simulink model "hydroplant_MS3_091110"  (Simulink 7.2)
settings: Solver=ode23tb  StartTime=0.0  StopTime=1000  MaxStep=0.1  RelTol=1e-4
undefined symbols (not defined in the file or in its folder): Blackbox_Base_sf, sigbuilder_block

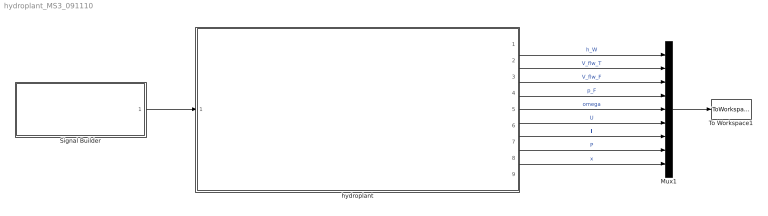
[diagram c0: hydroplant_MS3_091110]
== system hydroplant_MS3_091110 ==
  Mux1 : Mux  Inputs=9
  Signal Builder : Subsystem  Tag=STV Subsys  LoadFcn=sigbuilder_block('load');  StartFcn=sigbuilder_block('start');  StopFcn=sigbuilder_block('stop');  ClipboardFcn=sigbuilder_block('clipboard');
  To Workspace1 : ToWorkspace  VariableName=daten  SampleTime=-1  SaveFormat=Structure With Time
  hydroplant : Subsystem
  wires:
  Signal Builder/1(u) -> hydroplant/1(u)
  Mux1/1 -> To Workspace1/1
  hydroplant/1(h_W) -> Mux1/1  "h_W"
  hydroplant/2(V_flw_T) -> Mux1/2  "V_flw_T"
  hydroplant/3(V_flw_F) -> Mux1/3  "V_flw_F"
  hydroplant/4(p_F) -> Mux1/4  "p_F"
  hydroplant/5(omega) -> Mux1/5  "omega"
  hydroplant/6(U) -> Mux1/6  "U"
  hydroplant/7(I) -> Mux1/7  "I"
  hydroplant/8(P) -> Mux1/8  "P"
  hydroplant/9(x) -> Mux1/9  "x"

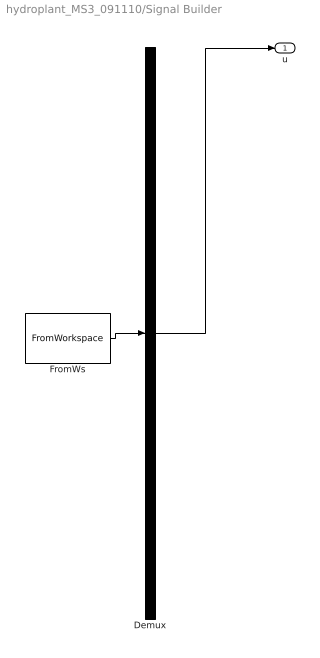
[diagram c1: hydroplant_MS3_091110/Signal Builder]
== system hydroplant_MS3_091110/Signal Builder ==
  Demux : Demux  Tag=STV Demux  Outputs=1
  FromWs : FromWorkspace  Tag=STV FromWs  VariableName=tuvar  SampleTime=0  SigBuilderData=DataTag0  VnvData=DataTag1
  u : Outport  Tag=STV Outport  OutDataType=sfix(16)  OutScaling=2^0
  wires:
  Demux/1 -> u/1
  FromWs/1 -> Demux/1

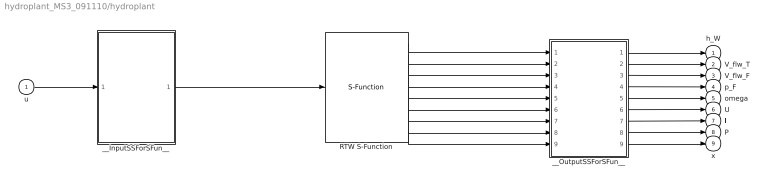
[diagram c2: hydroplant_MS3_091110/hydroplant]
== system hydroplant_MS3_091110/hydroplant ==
  u : Inport  OutDataType=sfix(16)  OutScaling=2^0
  RTW S-Function : S-Function  FunctionName=Blackbox_Base_sf  SFunctionModules=""  EnableBusSupport=off  mask{rtw_sf_name=Blackbox_Base_sf, showVar=off}
      mask prompts: rtw_sf_name "Generated S-function name (model_sf):"; showVar "Show module list"
      mask help: Real-Time Workshop generated S-function.
      mask init:
      | displist = '';
      | if ~strcmp(get_param(gcb, 'FunctionName'), rtw_sf_name);
      |   set_param(gcb, 'FunctionName', rtw_sf_name);
      | end
      | % Check if we are generating RTW code
      | rtw_mode = false;
      | if strcmpi(get_param(bdroot(gcb),'SimulationStatus'),'Initializing')
      | 	rtw_mode = strcmpi(get_param(bdroot(gcb),'BuildingRTWCode'),'on') && ...
      | 		~strcmpi(get_param(bdroot(gcb),'TargetStyle'),'SimulationTarget');
      | end
      | if showVar || rtw_mode
      | 	if exist('rtwsfunc') == 2 | exist('rtwsfunc') == 6
      | 		tmplist = rtwsfunc(rtw_sf_name,gcb);
      | 		tmplist = ['\nList of Modules:\n', tmplist];
      | 	elseif showVar
      | 		tmplist = '\nList of Modules:\nRTW not licensed\n';
      |  	end
      | end
      | if showVar
      |   displist = tmplist;
      | end
  __InputSSForSFun__ : Subsystem
  __OutputSSForSFun__ : Subsystem
  h_W : Outport  PortDimensions=1  SampleTime=[-1 0]  DataType=double  OutDataType=sfix(16)  OutScaling=2^0  OutDataTypeStr=double
  V_flw_T : Outport  Port=2  PortDimensions=1  SampleTime=[-1 0]  DataType=double  OutDataType=sfix(16)  OutScaling=2^0  OutDataTypeStr=double
  V_flw_F : Outport  Port=3  PortDimensions=1  SampleTime=[-1 0]  DataType=double  OutDataType=sfix(16)  OutScaling=2^0  OutDataTypeStr=double
  p_F : Outport  Port=4  PortDimensions=1  SampleTime=[-1 0]  DataType=double  OutDataType=sfix(16)  OutScaling=2^0  OutDataTypeStr=double
  omega : Outport  Port=5  PortDimensions=1  SampleTime=[-1 0]  DataType=double  OutDataType=sfix(16)  OutScaling=2^0  OutDataTypeStr=double
  U : Outport  Port=6  PortDimensions=1  SampleTime=[-1 0]  DataType=double  OutDataType=sfix(16)  OutScaling=2^0  OutDataTypeStr=double
  I : Outport  Port=7  PortDimensions=1  SampleTime=[-1 0]  DataType=double  OutDataType=sfix(16)  OutScaling=2^0  OutDataTypeStr=double
  P : Outport  Port=8  PortDimensions=1  SampleTime=[-1 0]  DataType=double  OutDataType=sfix(16)  OutScaling=2^0  OutDataTypeStr=double
  x : Outport  Port=9  PortDimensions=1  SampleTime=[-1 0]  DataType=double  OutDataType=sfix(16)  OutScaling=2^0  OutDataTypeStr=double
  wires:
  u/1 -> __InputSSForSFun__/1(u)
  __InputSSForSFun__/1(__UniqueOutportName__1__) -> RTW S-Function/1
  RTW S-Function/1 -> __OutputSSForSFun__/1(__UniqueInportName__1__)
  RTW S-Function/2 -> __OutputSSForSFun__/2(__UniqueInportName__2__)
  RTW S-Function/3 -> __OutputSSForSFun__/3(__UniqueInportName__3__)
  RTW S-Function/4 -> __OutputSSForSFun__/4(__UniqueInportName__4__)
  RTW S-Function/5 -> __OutputSSForSFun__/5(__UniqueInportName__5__)
  RTW S-Function/6 -> __OutputSSForSFun__/6(__UniqueInportName__6__)
  RTW S-Function/7 -> __OutputSSForSFun__/7(__UniqueInportName__7__)
  RTW S-Function/8 -> __OutputSSForSFun__/8(__UniqueInportName__8__)
  RTW S-Function/9 -> __OutputSSForSFun__/9(__UniqueInportName__9__)
  __OutputSSForSFun__/1(h_W) -> h_W/1
  __OutputSSForSFun__/2(V_flw_T) -> V_flw_T/1
  __OutputSSForSFun__/3(V_flw_F) -> V_flw_F/1
  __OutputSSForSFun__/4(p_F) -> p_F/1
  __OutputSSForSFun__/5(omega) -> omega/1
  __OutputSSForSFun__/6(U) -> U/1
  __OutputSSForSFun__/7(I) -> I/1
  __OutputSSForSFun__/8(P) -> P/1
  __OutputSSForSFun__/9(x) -> x/1

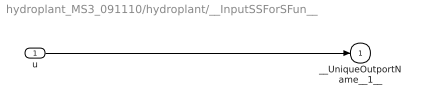
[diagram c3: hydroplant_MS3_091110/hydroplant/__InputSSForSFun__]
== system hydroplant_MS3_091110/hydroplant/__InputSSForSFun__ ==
  u : Inport  OutDataType=sfix(16)  OutScaling=2^0
  __UniqueOutportName__1__ : Outport  OutDataType=sfix(16)  OutScaling=2^0
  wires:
  u/1 -> __UniqueOutportName__1__/1

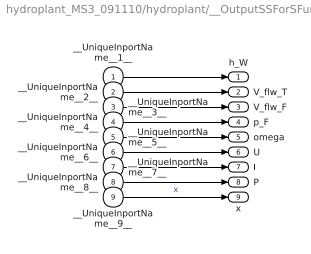
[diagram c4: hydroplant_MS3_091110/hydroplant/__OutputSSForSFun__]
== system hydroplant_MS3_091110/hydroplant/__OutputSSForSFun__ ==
  __UniqueInportName__1__ : Inport  OutDataType=sfix(16)  OutScaling=2^0
  __UniqueInportName__2__ : Inport  Port=2  OutDataType=sfix(16)  OutScaling=2^0
  __UniqueInportName__3__ : Inport  Port=3  OutDataType=sfix(16)  OutScaling=2^0
  __UniqueInportName__4__ : Inport  Port=4  OutDataType=sfix(16)  OutScaling=2^0
  __UniqueInportName__5__ : Inport  Port=5  OutDataType=sfix(16)  OutScaling=2^0
  __UniqueInportName__6__ : Inport  Port=6  OutDataType=sfix(16)  OutScaling=2^0
  __UniqueInportName__7__ : Inport  Port=7  OutDataType=sfix(16)  OutScaling=2^0
  __UniqueInportName__8__ : Inport  Port=8  OutDataType=sfix(16)  OutScaling=2^0
  __UniqueInportName__9__ : Inport  Port=9  OutDataType=sfix(16)  OutScaling=2^0
  h_W : Outport  PortDimensions=1  SampleTime=[-1 0]  DataType=double  OutDataType=sfix(16)  OutScaling=2^0  OutDataTypeStr=double
  V_flw_T : Outport  Port=2  PortDimensions=1  SampleTime=[-1 0]  DataType=double  OutDataType=sfix(16)  OutScaling=2^0  OutDataTypeStr=double
  V_flw_F : Outport  Port=3  PortDimensions=1  SampleTime=[-1 0]  DataType=double  OutDataType=sfix(16)  OutScaling=2^0  OutDataTypeStr=double
  p_F : Outport  Port=4  PortDimensions=1  SampleTime=[-1 0]  DataType=double  OutDataType=sfix(16)  OutScaling=2^0  OutDataTypeStr=double
  omega : Outport  Port=5  PortDimensions=1  SampleTime=[-1 0]  DataType=double  OutDataType=sfix(16)  OutScaling=2^0  OutDataTypeStr=double
  U : Outport  Port=6  PortDimensions=1  SampleTime=[-1 0]  DataType=double  OutDataType=sfix(16)  OutScaling=2^0  OutDataTypeStr=double
  I : Outport  Port=7  PortDimensions=1  SampleTime=[-1 0]  DataType=double  OutDataType=sfix(16)  OutScaling=2^0  OutDataTypeStr=double
  P : Outport  Port=8  PortDimensions=1  SampleTime=[-1 0]  DataType=double  OutDataType=sfix(16)  OutScaling=2^0  OutDataTypeStr=double
  x : Outport  Port=9  PortDimensions=1  SampleTime=[-1 0]  DataType=double  OutDataType=sfix(16)  OutScaling=2^0  OutDataTypeStr=double
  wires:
  __UniqueInportName__1__/1 -> h_W/1
  __UniqueInportName__2__/1 -> V_flw_T/1
  __UniqueInportName__3__/1 -> V_flw_F/1
  __UniqueInportName__4__/1 -> p_F/1
  __UniqueInportName__5__/1 -> omega/1
  __UniqueInportName__6__/1 -> U/1
  __UniqueInportName__7__/1 -> I/1
  __UniqueInportName__8__/1 -> P/1
  __UniqueInportName__9__/1 -> x/1  "x"
